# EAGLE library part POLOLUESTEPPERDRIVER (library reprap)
Pololu stepper driver based on the A4983.
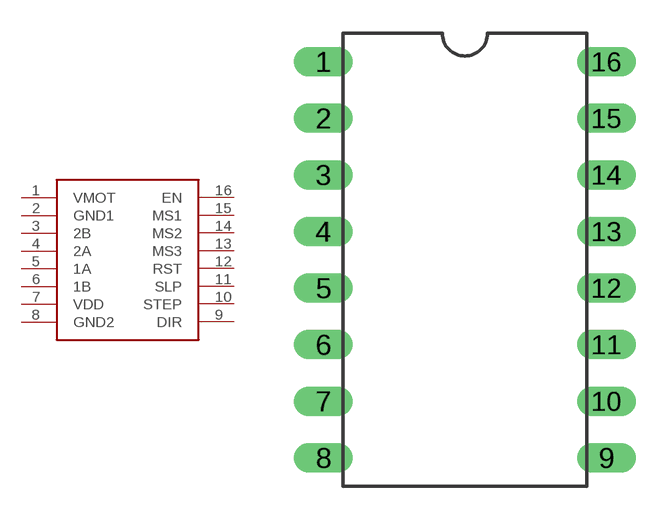
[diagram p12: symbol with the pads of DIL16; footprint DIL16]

Designator prefix -

## POLOLUESTEPPERDRIVER  [DIL16]
1  VMOT  pwr
2  GND1  pwr
3  2B  out
4  2A  out
5  1A  out
6  1B  out
7  VDD  pwr
8  GND2  pwr
9  DIR  in
10  STEP  in
11  SLP  in
12  RST  in
13  MS3  in
14  MS2  in
15  MS1  in
16  EN  in

## Footprint DIL16 (pad centres in mm)
drill 0.813 long: 1 -6.35,15.24; 2 -6.35,12.7; 3 -6.35,10.16; 4 -6.35,7.62; 5 -6.35,5.08; 6 -6.35,2.54; 7 -6.35,0; 8 -6.35,-2.54; 9 6.35,-2.54; 10 6.35,0; 11 6.35,2.54; 12 6.35,5.08; 13 6.35,7.62; 14 6.35,10.16; 15 6.35,12.7; 16 6.35,15.24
